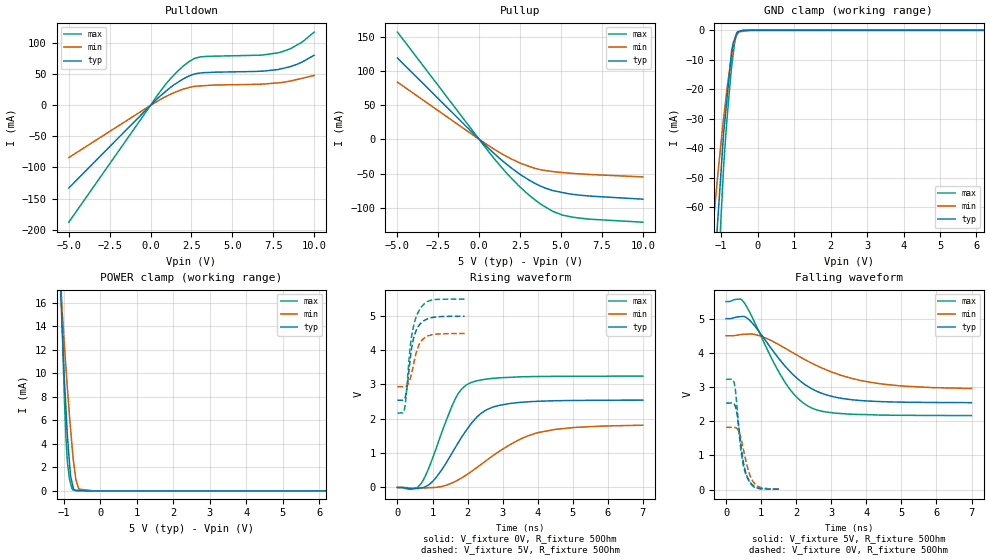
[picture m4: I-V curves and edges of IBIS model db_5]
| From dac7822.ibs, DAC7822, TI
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|   db_5 Model
[Model]   db_5
Model_type   I/O
Polarity   Non-Inverting
Enable   Active-Low
Vinl = 0.8
Vinh = 2.4
Vmeas = 2.5
Vref = 2.5
Cref = 2pF
Rref = 50
|   typ   min   max
|   (nom PVT)   (fast PVT)   (slow PVT)
|C_comp from frequency sweep method (F=83.3MHz)
|Average
|C_comp   3.122e-12   2.944e-12   3.147e-12
|ON state : BUFFER OUTPUT TURNED HIGH
|C_comp   3.479e-12   3.354e-12   3.682e-12
|OFF state: BUFFER IN HIGH IMPEDANCE
|C_comp   2.611e-12   2.533e-12   2.765e-12
|C_comp from LC tank measurement(L=1nH)
|Resonant Frequency(Hz)   3.360e+09   3.360e+09   3.250e+09
C_comp   2.246e-12   2.246e-12   2.401e-12
|ON state : BUFFER OUTPUT TURNED HIGH
|Resonant Frequency(Hz)   3.330e+09   3.330e+09   3.210e+09
|C_comp   2.287e-12   2.287e-12   2.461e-12
|OFF state: BUFFER IN HIGH IMPEDANCE
|Resonant Frequency(Hz)   3.360e+09   3.360e+09   3.250e+09
|C_comp   2.246e-12   2.246e-12   2.401e-12
| Where nom  PVT is Nominal Process, 5V, 25C
|   Fast PVT is Strong Process,  5.5V, -40C
|   Slow PVT is Weak Process,   4.5V, 125C
[Voltage Range]   5   4.5   5.5
|Ambient Temperature   25   125   -40
|Junction Temperature
[Temperature Range]   25   125   -40
[Pullup Reference]   5   4.5   5.5
[Pulldown Reference]   0   0   0
[Power Clamp Reference]   5   4.5   5.5
[GND Clamp Reference]   0   0   0
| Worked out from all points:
|   slope of the pulldown table from 0 to 0.75 V, typ, clamps not added: 40.5 ohm
|   slope of the pullup table from 0 to 0.75 V, typ, clamps not added: 43.9 ohm
|   GND clamp passes 1 mA (typ) near -0.57 V on its own axis
|   POWER clamp passes 1 mA (typ) near -0.79 V on its own axis
|   falling waveform, V_fixture 5V, R_fixture 50Ohm: 20-80 % time 1.28ns typ, 1.95ns min, 1.06ns max; typ from 5 V to 2.54 V
|   rising waveform, V_fixture 0V, R_fixture 50Ohm: 20-80 % time 993ps typ, 1.64ns min, 730ps max; typ from 0 V to 2.54 V
|   rising waveform, V_fixture 5V, R_fixture 50Ohm: 20-80 % time 219ps typ, 240ps min, 228ps max; typ from 2.54 V to 4.99 V
|   falling waveform, V_fixture 0V, R_fixture 50Ohm: 20-80 % time 217ps typ, 265ps min, 206ps max; typ from 2.53 V to 0.016 V
[Pulldown]
|   Voltage   I(typ)   I(min)   I(max)
-5V       -133mA     -84.08mA   -188.1mA
533.5mV   13.7mA     8.324mA    20.46mA
1.232V    29.19mA    18.02mA    43.36mA
2.024V    42.81mA    26.18mA    63.75mA
2.695V    50.5mA     30.52mA    75.6mA
3.08V     52.16mA    31.28mA    78.02mA
6.6V      54.7mA     33.96mA    80.62mA
7.788V    57.58mA    36.17mA    84.46mA
8.563V    62.39mA    39.12mA    91.26mA
9.29V     69.97mA    43.64mA    102.2mA
10V       80.59mA    48.07mA    117.8mA
[GND Clamp]
|   Voltage   I(typ)   I(min)   I(max)
-5V       -982mA     -674.9mA   -1.406A
-1.221V   -90.6mA    -66.19mA   -127mA
-1.1V     -65.8mA    -50.12mA   -90.39mA
-1.071V   -60.43mA   -46.31mA   -82.22mA
-1.006V   -48.51mA   -38.59mA   -64.21mA
-907.5mV  -31.78mA   -27.22mA   -41.56mA
-836mV    -22.66mA   -19.5mA    -29.52mA
-715mV    -7.22mA    -8.954mA   -12.54mA
-632.5mV  -3.028mA   -3.894mA   -4.348mA
-550mV    -502.2uA   -1.209mA   -721.2uA
-202.5mV  -3.002uA   -380nA     -1.463uA
10V       0A         0A         0A
[Pullup]
|   Voltage   I(typ)   I(min)   I(max)
-5V       119mA      83.73mA    156.9mA
0V        0A         0A         0A
968mV     -21.81mA   -15.17mA   -29.74mA
1.672V    -36.3mA    -24.98mA   -49.34mA
2.376V    -49.09mA   -33.36mA   -66.91mA
3.416V    -64.44mA   -42.48mA   -88.67mA
3.872V    -69.59mA   -44.91mA   -96.5mA
4.51V     -74.96mA   -47.06mA   -105.4mA
5.192V    -78.28mA   -48.72mA   -111.3mA
6.6V      -82.58mA   -51.1mA    -116.4mA
10V       -87.41mA   -54.87mA   -121.1mA
[POWER Clamp]
|   Voltage   I(typ)   I(min)   I(max)
-5V       357.8mA    285.4mA    439.7mA
-1.08V    16.44mA    17.01mA    18.13mA
-1.05V    14.24mA    15.58mA    14.65mA
-979mV    9.109mA    12.16mA    7.391mA
-940.5mV  6.891mA    10.42mA    4.45mA
-907.5mV  4.989mA    8.983mA    2.721mA
-820mV    1.395mA    5.456mA    708.2uA
-742.5mV  214.5uA    2.7mA      66.54uA
-670.5mV  19.13uA    973.8uA    60.09uA
-589.5mV  11.84uA    159.8uA    52.83uA
-202.5mV  0A         10.28nA    18.15uA
10V       0A         0A         0A
[Ramp]
R_load = 50
|   typ   min   max
dV/dt_r   1.52598/9.90689e-10   1.08808/1.63529e-09   1.94517/7.29369e-10
dV/dt_f   1.47343/1.28278e-09   0.925542/1.95177e-09   1.99992/1.05799e-09
[Falling Waveform]
V_fixture = 5V
V_fixture_min = 4.5V
V_fixture_max = 5.5V
R_fixture = 50Ohm
|   Time   V(typ)   V(min)   V(max)
0s        5V         4.5V       5.5V
407ps     5.059V     4.534V     5.573V
493ps     5.065V     4.542V     5.495V
811ps     4.794V     4.54V      4.896V
1.674ns   3.622V     4.14V      3.148V
2.04ns    3.241V     3.921V     2.677V
2.435ns   2.954V     3.702V     2.39V
3.135ns   2.7V       3.393V     2.237V
4.021ns   2.593V     3.156V     2.195V
6.999ns   2.544V     2.957V     2.167V
[Rising Waveform]
V_fixture = 0V
V_fixture_min = 0V
V_fixture_max = 0V
R_fixture = 50Ohm
|   Time   V(typ)   V(min)   V(max)
0s        1.902nV    2.65nV     1.631nV
462ps     -32.95mV   -27.2mV    -34.5mV
677ps     -12.49mV   -21.4mV    119.1mV
1.085ns   267.5mV    253.1uV    1.085V
1.634ns   1.135V     167.8mV    2.548V
1.827ns   1.46V      276.2mV    2.862V
2.078ns   1.825V     442.8mV    3.046V
2.696ns   2.33V      906.2mV    3.175V
3.919ns   2.506V     1.571V     3.23V
6.999ns   2.543V     1.813V     3.242V
[Rising Waveform]
V_fixture = 5V
V_fixture_min = 4.5V
V_fixture_max = 5.5V
R_fixture = 50Ohm
|   Time   V(typ)   V(min)   V(max)
0s        2.539V     2.936V     2.164V
156ps     2.542V     2.936V     2.174V
205ps     2.588V     2.936V     2.305V
271ps     2.896V     2.962V     2.942V
339ps     3.506V     3.086V     3.838V
391ps     3.958V     3.268V     4.313V
484ps     4.431V     3.702V     4.801V
620ps     4.728V     4.166V     5.16V
975ps     4.946V     4.446V     5.46V
1.917ns   4.987V     4.487V     5.487V
[Falling Waveform]
V_fixture = 0V
V_fixture_min = 0V
V_fixture_max = 0V
R_fixture = 50Ohm
|   Time   V(typ)   V(min)   V(max)
0s        2.532V     1.822V     3.226V
231ps     2.5V       1.822V     3.117V
306ps     2.248V     1.792V     2.473V
381ps     1.657V     1.653V     1.555V
440ps     1.16V      1.426V     1.018V
533ps     596mV      983.9mV    540.6mV
623ps     324.5mV    602.4mV    312.1mV
755ps     135.4mV    258.8mV    111.7mV
898ps     50.56mV    105.2mV    38.81mV
1.553ns   15.75mV    14.59mV    18.33mV
